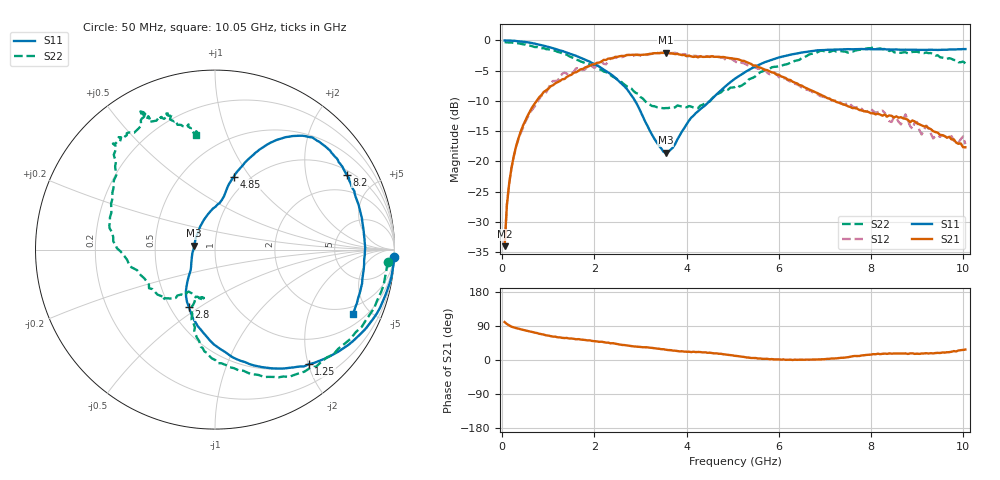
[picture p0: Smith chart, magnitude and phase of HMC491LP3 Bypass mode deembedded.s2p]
!Hittite Microwave Corporation
!12 Elizabeth Drive
!Chelmsford, MA 01824
!Tel: 978-250-3343
!Fax: 978-250-3373
!Device: HMC491LP3, 3.4-3.8 GHz, GaAs MMIC Low Noise Amplifier with Bypass Mode in leadless SMT package
!Misc: Bypass Mode, Room
# MHZ S MA R 50
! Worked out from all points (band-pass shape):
!   201 points, 50 MHz to 10.05 GHz, reference 50 ohm
!   highest |S21| = -2.06 dB at 3.55 GHz (marker M1); lowest = -34.0 dB at 50 MHz (marker M2)
!   |S21| within 3 dB of the highest: 1.648 GHz to 5.784 GHz (4.135 GHz wide, 111 % of centre)
!   lowest |S11| = -18.6 dB at 3.55 GHz (marker M3), VSWR 1.27, Z = 39.6 + j1.71 ohm
!   |S11| at or under -10 dB: 2.882 GHz to 4.504 GHz (1.623 GHz wide, 43.9 % of centre)
!   |S22| runs from -11.2 to -0.3 dB; largest |S21 - S12| = 0.064
!   S11 on the Smith chart (normalised r, x): 50 MHz: 2, -50; 1.25 GHz: 0.50, -2.01; 2.8 GHz: 0.62, -0.45; 4.85 GHz: 0.85, +0.84; 8.2 GHz: 1.17, +3.40; 10.05 GHz: 1.53, -3.90
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50  0.998 -2.3  0.02 100.2  0.02 102.3  0.965 -4.2
100  0.998 -4.3  0.044 94.9  0.044 94.7  0.962 -6.8
150  0.996 -6.5  0.066 91.2  0.067 91.0  0.96 -9.3
400  0.978 -17.2  0.177 81.0  0.172 80.5  0.937 -22.3
850  0.914 -35.4  0.354 68.2  0.349 69.7  0.861 -47.1
1250  0.825 -50.8  0.461 59.8  0.496 62.0  0.795 -63.5
1750  0.705 -68.2  0.581 53.4  0.568 50.4  0.66 -82.9
2350  0.527 -90.9  0.708 44.0  0.708 47.7  0.516 -99.9
2800  0.352 -114.3  0.759 36.6  0.736 36.9  0.401 -108.9
3400  0.135 -162.5  0.784 29.7  0.784 30.3  0.278 -105.3
3550  0.118 169.6  0.789 27.1  0.796 28.1  0.276 -103.6
4250  0.26 84.4  0.724 21.2  0.736 19.8  0.276 -122.1
4850  0.42 75.5  0.722 14.4  0.691 12.3  0.402 -136.0
5050  0.483 72.4  0.703 10.9  0.671 9.2  0.412 -147.7
5850  0.691 61.2  0.544 2.4  0.537 5.4  0.6 168.5
6750  0.819 49.9  0.38 1.2  0.369 2.3  0.779 135.7
8200  0.844 29.7  0.244 15.5  0.256 15.3  0.859 117.9
8400  0.841 26.3  0.24 17.5  0.215 12.9  0.816 116.5
8750  0.838 17.3  0.225 17.5  0.245 18.0  0.797 112.3
9100  0.835 7.3  0.199 17.1  0.167 18.5  0.79 109.2
9200  0.835 4.2  0.195 18.0  0.198 23.2  0.794 108.2
10050  0.847 -25.2  0.131 27.6  0.139 22.5  0.646 99.4
